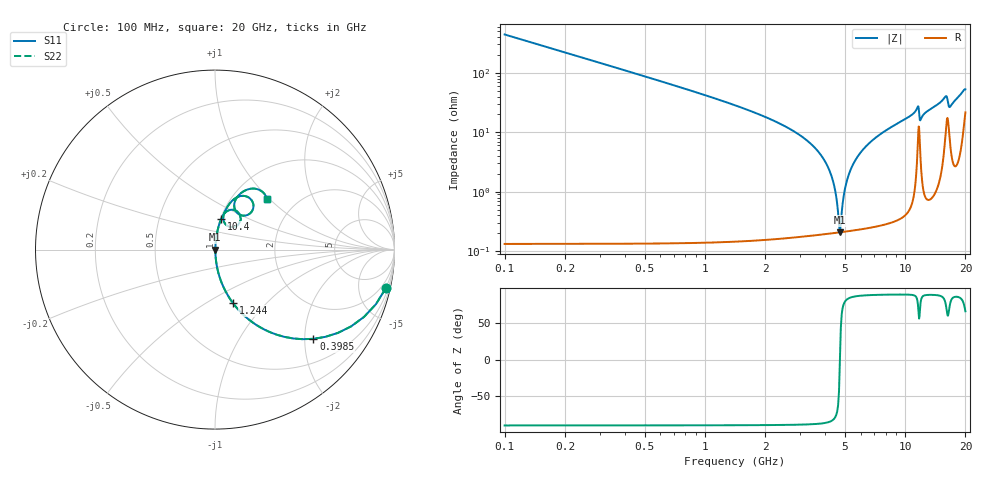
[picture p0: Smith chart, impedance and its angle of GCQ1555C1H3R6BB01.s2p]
!Murata Part Number: GCQ1555C1H3R6BB01
!These Parameters are Measured in Series Mode Connection
!Data Generated on Mar 13, 2026
!  o--ll--o
!Port1  Port2
!  o------o
!Operation Temp=25[degC], DC Bias Voltage=0[V]
!Freq. Start=100[MHz] Stop=20[GHz] 401[Steps]
# Hz S RI R 50
!Freq.(Hz) S11(Real) S11(Imag) S21(Real) S21(Imag) S12(Real) S12(Imag) S22(Real) S22(Imag)
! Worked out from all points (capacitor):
!   401 points, 100 MHz to 20 GHz, reference 50 ohm
!   read as one part in series: C = 3.6 pF near 199.5 MHz
!   lowest |Z| = 208 mohm at 4.727 GHz (marker M1)
!   series resonance near 4.725 GHz, so ESL is about 320 pH
!   S11 on the Smith chart (normalised r, x): 100 MHz: 1.00, -8.84; 398.5 MHz: 1.00, -2.20; 1.244 GHz: 1.00, -0.66; 10.4 GHz: 1.01, +0.36; 20 GHz: 1.43, +0.96
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1e8  0.9512 -0.2152  0.0488 0.2152  0.0488 0.2152  0.9512 -0.2152
3.985e8  0.5481 -0.4971  0.4519 0.4971  0.4519 0.4971  0.5481 -0.4971
7.4675e8  0.2505 -0.4321  0.7495 0.4321  0.7495 0.4321  0.2505 -0.4321
1.24425e9  0.0997 -0.2974  0.9003 0.2974  0.9003 0.2974  0.0997 -0.2974
3.43325e9  0.00551 -0.0606  0.9945 0.0606  0.9945 0.0606  0.00551 -0.0606
4.279e9  0.00234 -0.0186  0.9977 0.0186  0.9977 0.0186  0.00234 -0.0186
4.478e9  0.00213 -0.0101  0.9979 0.0101  0.9979 0.0101  0.00213 -0.0101
4.62725e9  0.00207 -0.00393  0.9979 0.00393  0.9979 0.00393  0.00207 -0.00393
4.72675e9  0.00207 6.84e-05  0.9979 -6.84e-05  0.9979 -6.84e-05  0.00207 6.84e-05
5.02525e9  0.00227 0.0116  0.9977 -0.0116  0.9977 -0.0116  0.00227 0.0116
5.3735e9  0.00279 0.0243  0.9972 -0.0243  0.9972 -0.0243  0.00279 0.0243
5.92075e9  0.00416 0.043  0.9958 -0.043  0.9958 -0.043  0.00416 0.043
6.7665e9  0.00736 0.0695  0.9926 -0.0695  0.9926 -0.0695  0.00736 0.0695
1.005e10  0.0313 0.1624  0.9687 -0.1624  0.9687 -0.1624  0.0313 0.1624
1.039825e10  0.0357 0.1731  0.9643 -0.1731  0.9643 -0.1731  0.0357 0.1731
1.15425e10  0.1044 0.2214  0.8956 -0.2214  0.8956 -0.2214  0.1044 0.2214
1.19405e10  0.0568 0.1434  0.9432 -0.1434  0.9432 -0.1434  0.0568 0.1434
1.338325e10  0.063 0.2282  0.937 -0.2282  0.937 -0.2282  0.063 0.2282
1.59205e10  0.1891 0.2895  0.8109 -0.2895  0.8109 -0.2895  0.1891 0.2895
1.67165e10  0.1184 0.2104  0.8816 -0.2104  0.8816 -0.2104  0.1184 0.2104
1.89055e10  0.183 0.3355  0.817 -0.3355  0.817 -0.3355  0.183 0.3355
2e10  0.2887 0.2814  0.7113 -0.2814  0.7113 -0.2814  0.2887 0.2814
